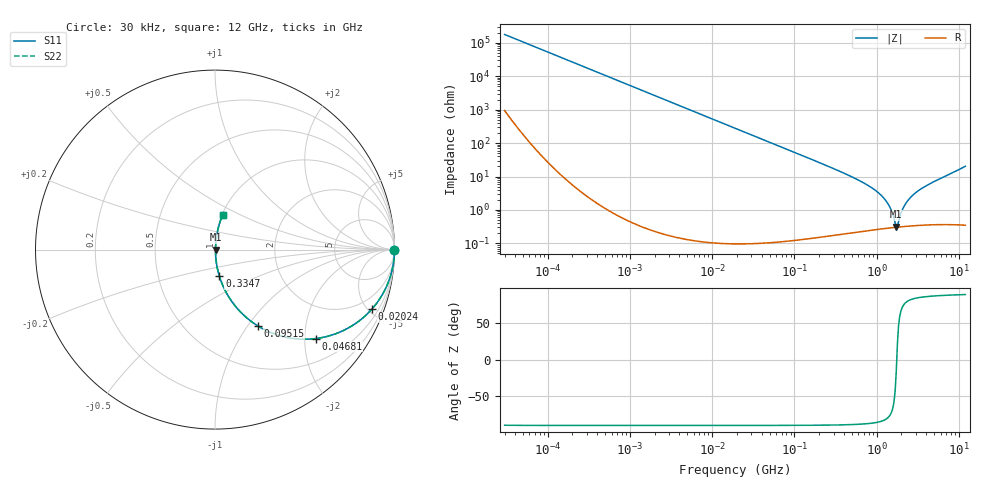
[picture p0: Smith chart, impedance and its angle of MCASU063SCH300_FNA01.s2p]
! MCASU063SCH300_FNA01  S-PARAMETER MODEL  ( General Type )
! Model Generated by TAIYO YUDEN Corporation (http://www.ty-top.com)
! Version 1.0
! TAIYO YUDEN Control No. 130801
! Copyright(c) 2013 TAIYO YUDEN CO.,LTD. All Rights Reserved.
! Product Description (link to TY-COMPAS)
! https://ds.yuden.co.jp/TYCOMPAS/or/detail?pn=MCASU063SCH300JFNA01&u=M
! Products Name : Multilayer Ceramic Capacitors
! Characteristics :
!  Capacitance : 30 pF , Rated Voltage : 50V , TCC : CH / C0H
!  Case Size : 0.6 x 0.3 / 0.024 x 0.012 [mm/inch] , Thickness : 0.3 / 0.012 [mm/inch]
!  (Conditions: Temperature = 25 degC , DC Bias Current/Voltage = 0A / 0V)
! External Node Assignments :
!  1  o---| |---o  2
! GND o---------o GND
! Frequency Range : 0.03MHz  -  12000MHz  [ 401 STEP ]
# MHz S RI R 50
! Freq[MHz].  S11 Real  S11 Imag  S21 Real  S21 Imag  S12 Real  S12 Imag  S22 Real  S22 Imag
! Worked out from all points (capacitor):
!   401 points, 30 kHz to 12 GHz, reference 50 ohm
!   read as one part in series: C = 29.9 pF near 32 kHz
!   lowest |Z| = 316 mohm at 1.733 GHz (marker M1)
!   series resonance near 1.757 GHz, so ESL is about 270 pH
!   S11 on the Smith chart (normalised r, x): 30 kHz: open; 20.24 MHz: 1.00, -5.26; 46.81 MHz: 1.00, -2.27; 95.15 MHz: 1.00, -1.11; 334.7 MHz: 1.00, -0.31; 12 GHz: 1.01, +0.40
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0.03  1 -0.000564  3.3e-06 0.000564  3.3e-06 0.000564  1 -0.000564
0.260295  1 -0.00489  2.47e-05 0.00489  2.47e-05 0.00489  1 -0.00489
2.258455  0.9982 -0.0424  0.0018 0.0424  0.0018 0.0424  0.9982 -0.0424
7.211021  0.9819 -0.1331  0.0181 0.1331  0.0181 0.1331  0.9819 -0.1331
18.97367  0.887 -0.3164  0.113 0.3164  0.113 0.3164  0.887 -0.3164
20.23772  0.8734 -0.3323  0.1266 0.3323  0.1266 0.3323  0.8734 -0.3323
46.80535  0.5632 -0.4955  0.4368 0.4955  0.4368 0.4955  0.5632 -0.4955
95.14999  0.2375 -0.4245  0.7625 0.4245  0.7625 0.4245  0.2375 -0.4245
164.6252  0.0941 -0.2897  0.9059 0.2897  0.9059 0.2897  0.0941 -0.2897
334.6645  0.0246 -0.1491  0.9754 0.1491  0.9754 0.1491  0.0246 -0.1491
598.0015  0.0083 -0.0778  0.9917 0.0778  0.9917 0.0778  0.0083 -0.0778
909.4299  0.00434 -0.0426  0.9957 0.0426  0.9957 0.0426  0.00434 -0.0426
1177.092  0.00334 -0.0248  0.9967 0.0248  0.9967 0.0248  0.00334 -0.0248
1428.372  0.00303 -0.0126  0.997 0.0126  0.997 0.0126  0.00303 -0.0126
1678.29  0.00301 -0.00282  0.997 0.00282  0.997 0.00282  0.00301 -0.00282
1733.294  0.00302 -0.000875  0.997 0.000875  0.997 0.000875  0.00302 -0.000875
1848.769  0.00308 0.00324  0.9969 -0.00324  0.9969 -0.00324  0.00308 0.00324
2036.564  0.00322 0.00899  0.9968 -0.00899  0.9968 -0.00899  0.00322 0.00899
2243.435  0.00343 0.0147  0.9966 -0.0147  0.9966 -0.0147  0.00343 0.0147
2998.885  0.00446 0.0327  0.9955 -0.0327  0.9955 -0.0327  0.00446 0.0327
4710.119  0.00781 0.0648  0.9922 -0.0648  0.9922 -0.0648  0.00781 0.0648
12000  0.0425 0.1932  0.9575 -0.1932  0.9575 -0.1932  0.0425 0.1932
